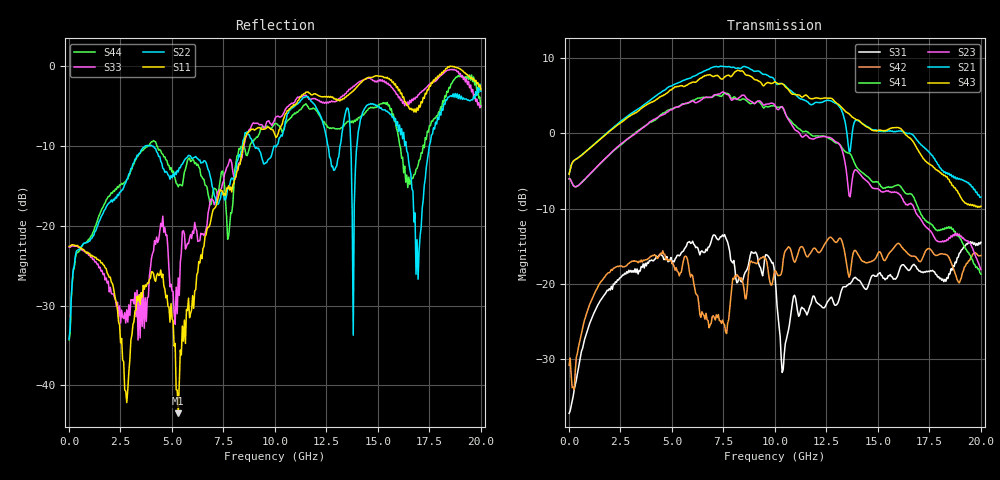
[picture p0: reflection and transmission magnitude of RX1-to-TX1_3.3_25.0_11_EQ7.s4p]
!Agilent Technologies,N5225A,MY51451112,A.09.50.13
!Agilent N5225A: A.09.50.13
!Date: Wednesday, January 31, 2018 11:04:14
!Correction: S11(Full 4 Port(1,2,3,4))
!S12(Full 4 Port(1,2,3,4))
!S13(Full 4 Port(1,2,3,4))
!S14(Full 4 Port(1,2,3,4))
!S21(Full 4 Port(1,2,3,4))
!S22(Full 4 Port(1,2,3,4))
!S23(Full 4 Port(1,2,3,4))
!S24(Full 4 Port(1,2,3,4))
!S31(Full 4 Port(1,2,3,4))
!S32(Full 4 Port(1,2,3,4))
!S33(Full 4 Port(1,2,3,4))
!S34(Full 4 Port(1,2,3,4))
!S41(Full 4 Port(1,2,3,4))
!S42(Full 4 Port(1,2,3,4))
!S43(Full 4 Port(1,2,3,4))
!S44(Full 4 Port(1,2,3,4))
!S4P File: Measurements: <S11,S12,S13,S14>,
!<S21,S22,S23,S24>,
!<S31,S32,S33,S34>,
!<S41,S42,S43,S44>:
# Hz S  RI  R 50
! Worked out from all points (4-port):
!   401 points, 10 MHz to 20 GHz, reference 50 ohm
!   strongest paths, dB at 10 MHz, 5.008 GHz, 10.01 GHz, 15 GHz, 20 GHz:
!     S43: -5.5, 5.8, 6.8, 0.4, -9.7
!     S21: -5.4, 6.3, 6.9, 0.4, -8.5
!     S23: -6.1, 3.1, 3.7, -7.4, -18.1
!     S41: -6.1, 3.2, 3.6, -6.5, -18.7
!     S42: -30.8, -17.3, -18.2, -15.9, -16.2
!     S31: -37.2, -17.3, -19.0, -18.7, -14.5
!   lowest |S11| = -43.5 dB at 5.307 GHz (marker M1), VSWR 1.01, Z = 49.3 - j0.0448 ohm
!   |S11| at or under -10 dB: start of sweep to 8.454 GHz
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1e7  -0.0744 -0.00266  0.000173 0.000507  0.0137 0.000389  -0.000448 0.000553
     0.5361 0.0105  -0.0131 0.0144  -0.4975 0.000555  0.0264 0.012
     0.0139 0.000379  -0.000289 0.000481  -0.0734 -0.00382  -0.000268 0.000942
     -0.4978 0.00152  0.0263 0.012  0.5335 0.00969  -0.0129 0.0143
5.30735e9  -0.00666 -0.000454  0.0285 -0.00433  0.0986 0.1377  0.0294 -0.014
           -0.936 -1.938  0.1252 -0.1784  0.8816 1.201  0.1226 0.00671
           0.0919 0.125  0.0328 -0.00109  0.0368 0.0295  0.0404 -0.0103
           1.196 0.9088  0.1187 0.0144  -1.538 -1.332  0.0641 -0.1638
7.10645e9  -0.0219 0.1286  0.016 -0.0174  0.1318 0.0775  0.00469 -0.0327
           -2.753 0.2076  0.1184 -0.092  1.744 -0.4424  0.0448 0.0269
           0.1731 0.1173  0.025 -0.0228  0.0115 0.1405  0.0152 -0.0451
           1.408 -1.1  0.0575 -0.00518  -2.025 1.299  0.1035 -0.136
8.755625e9  0.00999 0.3936  0.0111 -0.0107  0.1029 0.0877  -0.00642 -0.0147
            -0.7043 2.595  -0.1023 0.3578  0.164 -1.645  0.0224 0.1346
            0.1131 0.0876  0.00397 -0.0243  0.0534 0.3994  -0.0129 -0.0267
            -0.5824 -1.471  -0.0215 0.1288  0.6743 2.31  0.2209 0.2087
1.04048e10  0.1127 0.4501  -0.0223 -0.0474  0.0218 -0.0107  -0.0542 -0.024
            1.572 1.402  0.2805 0.2725  -1.307 -0.662  0.0205 0.1562
            -0.0266 0.00545  -0.0301 -0.0458  0.2017 0.4615  -0.0591 -0.0289
            -1.446 0.109  0.0562 0.1336  2.088 0.2703  0.3873 -0.0905
1.270365e10  0.2743 0.5867  -0.0374 -0.00979  0.0206 0.0717  -0.0311 0.00766
             1.393 -0.8659  0.1581 0.2103  -0.6608 0.6558  0.1818 0.1031
             0.023 0.0777  -0.0308 -0.0104  0.3944 0.4485  -0.0425 -0.0019
             -0.1152 0.9029  0.1785 0.0994  0.3451 -1.669  0.2479 -0.3282
2e10  0.7114 0.0659  0.0231 0.0349  -0.0787 0.1636  0.0347 0.0207
      -0.0186 0.3762  0.6934 0.0755  0.0456 -0.116  0.1535 0.0419
      -0.0796 0.1713  0.00639 0.0478  0.5645 -0.0274  0.0477 0.0205
      -0.0915 -0.0718  0.1471 0.0461  0.2989 0.1343  -0.1522 -0.5322
